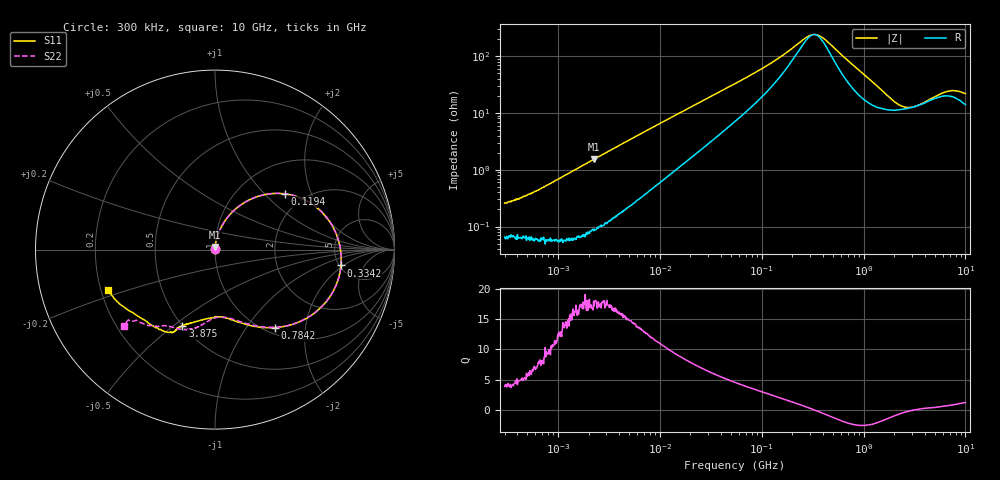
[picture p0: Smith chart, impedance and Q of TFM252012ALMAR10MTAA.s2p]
! S-Parameter Data Generated by TDK Corporation
! Copyright(C) 2019 TDK Corporation.
! All Rights Reserved.
! TDK P/N: TFM252012ALMAR10MTAA (Inductor)
! Property: L=100nH at 1MHz
! Size(LxWxT):
! Model Type: s2p (Touchstone File Format Version 1.0)
! Frequency: DC=Yes Start=0.3MHz Stop=10000MHz 802points Log-sweep
! Model Generated on Sep. 23, 2019
! Port Assignments:
!  1 ---@@@--- 2
! Applicable Conditions:
!  Temperature = 25 degC
!  DC Bias Current = 0 A
!  Small Signal Operation
! Terms and conditions regarding TDK Simulation Models
! (1)This simulation model is being provided solely for informational purposes. Please refer to the specifications of the products in terms of detailed characteristics of such products.
! (2)In no event shall TDK Corporation of any of its subsidiaries be liable for any loss or damage arising, directly or indirectly,
!  From any information contained in this simulation model, including, but not limited to loss or damages arising from any inaccuracies, omissions or errors in connection with such information.
! (3)Any and all copyrights on this simulation model are owned by TDK Corporation.
!  Duplication or redistribution of this simulation model without prior written permission from TDK Corporation is prohibited.
! (4)This simulation model is subject to any modification or change without any prior notice.
! (5)Neither TDK Corporation nor any of its subsidiaries shall make any warranty, express or implied,
!  Including but not limited to the correctness, implied warranties of merchantability and fitness for a particular purpose with respect to this simulation models.
! (6)The use of this simulation model shall be deemed to have consented to the terms and conditions hereof.
# Hz S MA R 50
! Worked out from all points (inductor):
!   801 points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, 300 kHz to 10 GHz, reference 50 ohm
!   read as one part in series: L = 118 nH near 318.3 kHz
!   highest Q = 17.8 at 2.244 MHz (marker M1), where L = 108 nH
!   self-resonance near 326.1 MHz
!   S11 on the Smith chart (normalised r, x): 300 kHz: 1.00, +0.01; 119.4 MHz: 1.60, +1.32; 334.2 MHz: 5.16, -1.82; 784.2 MHz: 1.10, -1.37; 3.875 GHz: 0.50, -0.54; 10 GHz: 0.23, -0.17
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300000  0.003902 85.9  0.9989 -0.1  0.9987 -0.1  0.003725 90.8
428090  0.004124 84.6  0.999 -0.1  0.9991 -0.1  0.004103 85.9
671858  0.005065 84.6  0.9993 -0.2  0.9993 -0.2  0.005189 85.4
1713600  0.01169 86.5  0.9991 -0.7  0.9991 -0.7  0.01175 87.0
2243505  0.01519 86.2  0.9988 -0.9  0.999 -0.9  0.01518 86.7
9671944  0.06122 81.1  0.9923 -3.6  0.9928 -3.6  0.06126 81.1
2.693747e7  0.1572 72.0  0.964 -9.4  0.9643 -9.4  0.1572 72.0
5.477226e7  0.2866 60.1  0.8966 -17.1  0.8968 -17.1  0.2866 60.1
1.19394e8  0.4975 38.6  0.7016 -29.4  0.7017 -29.4  0.4976 38.7
1.923314e8  0.6278 19.9  0.489 -33.4  0.4891 -33.4  0.6277 20.0
3.126428e8  0.7041 -3.6  0.2964 -9.2  0.2965 -9.2  0.7048 -3.5
3.342219e8  0.7071 -7.2  0.2933 -1.9  0.2934 -1.9  0.7079 -7.0
4.269249e8  0.6961 -20.3  0.357 19.3  0.3571 19.3  0.6975 -20.0
5.344909e8  0.6563 -32.7  0.4771 25.0  0.4773 25.0  0.6578 -32.3
7.84152e8  0.5473 -52.7  0.6709 18.3  0.671 18.3  0.5496 -51.9
1.196827e9  0.4293 -71.1  0.7921 4.6  0.7922 4.6  0.4332 -69.3
1.767019e9  0.3751 -85.8  0.8267 -9.0  0.8267 -9.0  0.3806 -82.3
2.568366e9  0.3934 -99.0  0.8083 -22.7  0.8083 -22.7  0.3952 -94.4
3.874538e9  0.4635 -113.1  0.7417 -38.3  0.7418 -38.3  0.4614 -105.6
6.495326e9  0.5363 -122.1  0.6342 -60.9  0.6342 -61.0  0.5139 -124.2
8.434726e9  0.5747 -141.7  0.5535 -77.5  0.5527 -77.6  0.5869 -137.5
1e10  0.6357 -159.5  0.4902 -87.0  0.4908 -87.1  0.6597 -140.1
